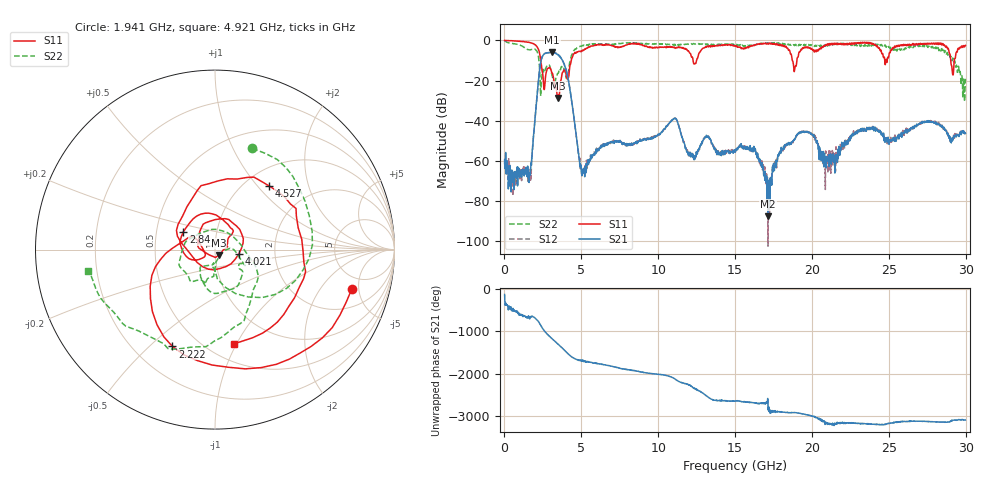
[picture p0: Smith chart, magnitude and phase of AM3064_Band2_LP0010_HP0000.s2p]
# Hz S DB R 50.0
!freq dBS11 angS11 dBS21 angS21 dBS12 angS12 dBS22 angS22
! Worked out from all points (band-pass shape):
!   1600 points, 10 MHz to 29.98 GHz, reference 50 ohm
!   highest |S21| = -5.90 dB at 3.103 GHz (marker M1); lowest = -87.7 dB at 17.14 GHz (marker M2)
!   |S21| within 3 dB of the highest: 2.42 GHz to 3.692 GHz (1.271 GHz wide, 41.6 % of centre)
!   lowest |S11| = -28.7 dB at 3.478 GHz (marker M3), VSWR 1.08, Z = 52.1 - j3.07 ohm
!   |S11| at or under -10 dB: 2.368 GHz to 4.343 GHz (1.975 GHz wide, 58.9 % of centre); 18.73 GHz to 19.02 GHz (293.9 MHz wide, 1.56 % of centre); 29.03 GHz to 29.26 GHz (229 MHz wide, 0.786 % of centre)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
!   |S22| runs from -30.4 to -0.2 dB; largest |S21 - S12| = 0.019
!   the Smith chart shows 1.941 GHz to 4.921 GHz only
!   S11 on the Smith chart (normalised r, x): 1.941 GHz: 3.58, -4.20; 2.222 GHz: 0.36, -0.59; 2.84 GHz: 0.69, +0.14; 4.021 GHz: 1.30, -0.07; 4.527 GHz: 1.28, +1.16; 4.921 GHz: 0.66, -0.98
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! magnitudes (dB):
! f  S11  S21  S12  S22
! 10 MHz  0.0  -59.7  -61.8  -0.2
! 1.603 GHz  -1.0  -70.8  -66.5  -4.6
! 1.941 GHz  -2.0  -43.2  -43.4  -4.4
! 2.222 GHz  -4.6  -19.2  -19.1  -8.5
! 2.84 GHz  -13.9  -6.2  -6.1  -12.4
! 3.103 GHz  -16.6  -5.9  -6.1  -17.5
! 3.478 GHz  -28.7  -7.0  -7.2  -16.5
! 4.021 GHz  -17.4  -15.2  -15.2  -18.9
! 4.527 GHz  -6.6  -38.9  -38.9  -5.0
! 4.921 GHz  -5.4  -61.3  -63.5  -2.9
! 5.015 GHz  -5.5  -66.1  -66.5  -2.9
! 10 GHz  -3.5  -47.2  -46.8  -1.8
! 15 GHz  -2.6  -55.6  -54.7  -1.9
! 16.26 GHz  -2.4  -53.4  -54.5  -2.4
! 17.14 GHz  -1.6  -87.7  -102.5  -1.4
! 18.15 GHz  -2.8  -52.8  -53.4  -2.0
! 19.99 GHz  -4.2  -46.7  -46.8  -2.2
! 20.89 GHz  -2.1  -58.0  -55.1  -2.8
! 25 GHz  -8.0  -50.3  -49.4  -3.0
! 28.56 GHz  -2.1  -43.3  -43.7  -4.8
! 29.18 GHz  -17.2  -49.2  -48.5  -8.9
! 29.98 GHz  -2.4  -46.3  -46.2  -19.1
